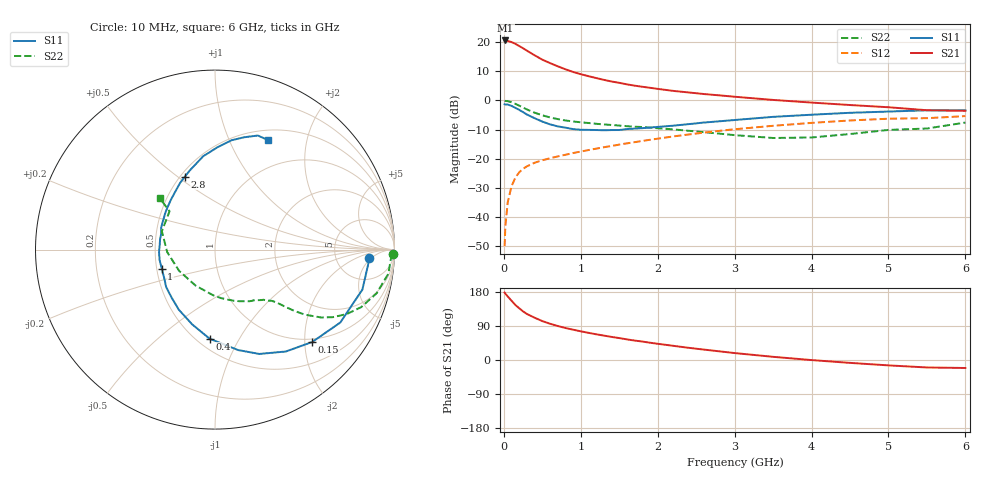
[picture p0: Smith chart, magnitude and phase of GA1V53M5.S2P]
! Infineon Technologies  Discrete & RF Semiconductors
! BF775
! Si NPN RF Bipolar Junction Transistor in SOT23
! VCE = 1.5 V  IC = 3.5 mA
! Common Emitter S-Parameters:  May  1996
# GHz  S  MA  R  50
!  f  S11  S21  S12  S22
! GHz  MAG  ANG  MAG  ANG  MAG  ANG  MAG  ANG
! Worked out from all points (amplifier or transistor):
!   36 points, 10 MHz to 6 GHz, reference 50 ohm
!   highest |S21| = 20.6 dB at 20 MHz (marker M1)
!   |S21| within 3 dB of that: start of sweep to 269.6 MHz
!   unconditionally stable (mu >= 1): 871.5 MHz to 4.679 GHz; 5.009 GHz to end of sweep
!   at 250 MHz: K = 0.40, MSG = 20.7 dB, |S12| = -23.4 dB
!   at 1.4 GHz: K = 1.16, MAG = 8.6 dB, |S12| = -15.6 dB
!   at 6 GHz: K = 1.01, MAG = 0.2 dB, |S12| = -5.4 dB
!   S11 on the Smith chart (normalised r, x): 10 MHz: 12, -4; 150 MHz: 0.93, -2.17; 400 MHz: 0.58, -0.76; 1 GHz: 0.53, -0.12; 2.8 GHz: 0.53, +0.53; 6 GHz: 0.62, +1.40
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0.01  0.8617 -3.1  10.6 177.8  0.0032 89.4  0.9919 -1.5
0.02  0.8563 -6.1  10.67 174.9  0.007 87.9  0.9809 -3.1
0.05  0.8509 -15.2  10.46 167.8  0.0179 81.9  0.9753 -7.9
0.1  0.8077 -30.2  10.01 156.4  0.0341 73.7  0.9329 -15.1
0.15  0.7474 -43.5  9.337 145.1  0.0476 67.0  0.8753 -21.5
0.2  0.6914 -55.2  8.564 136.5  0.059 62.4  0.8166 -26.1
0.25  0.6316 -67.0  7.833 128.2  0.0674 57.8  0.7574 -29.8
0.3  0.5745 -77.0  7.135 121.5  0.0746 55.0  0.7019 -32.6
0.4  0.4971 -93.5  5.938 111.6  0.0858 51.3  0.6181 -35.9
0.5  0.4352 -107.1  5.003 102.7  0.0947 49.5  0.5578 -37.7
0.6  0.3909 -121.0  4.37 95.7  0.1024 48.6  0.5134 -38.9
0.7  0.3602 -132.3  3.853 89.7  0.1102 48.6  0.4801 -39.8
0.8  0.3425 -142.7  3.426 84.5  0.1175 48.6  0.4548 -40.6
1  0.315 -160.4  2.822 75.7  0.1334 49.1  0.4234 -42.3
1.1  0.314 -169.3  2.608 71.7  0.1416 49.2  0.4114 -43.7
1.6  0.324 157.6  1.889 54.4  0.1845 49.4  0.3629 -50.8
2.2  0.3699 131.9  1.461 37.5  0.2421 46.6  0.32 -64.1
2.8  0.44 112.4  1.225 22.9  0.3017 41.4  0.271 -83.5
3.5  0.5243 97.2  1.022 8.4  0.3686 33.4  0.2279 -118.3
4.5  0.6155 81.5  0.836 -7.6  0.4547 20.4  0.2666 -177.0
5.5  0.6789 69.4  0.681 -19.7  0.4981 5.9  0.3312 139.9
6  0.678 64.3  0.666 -21.1  0.54 1.8  0.4189 137.1
